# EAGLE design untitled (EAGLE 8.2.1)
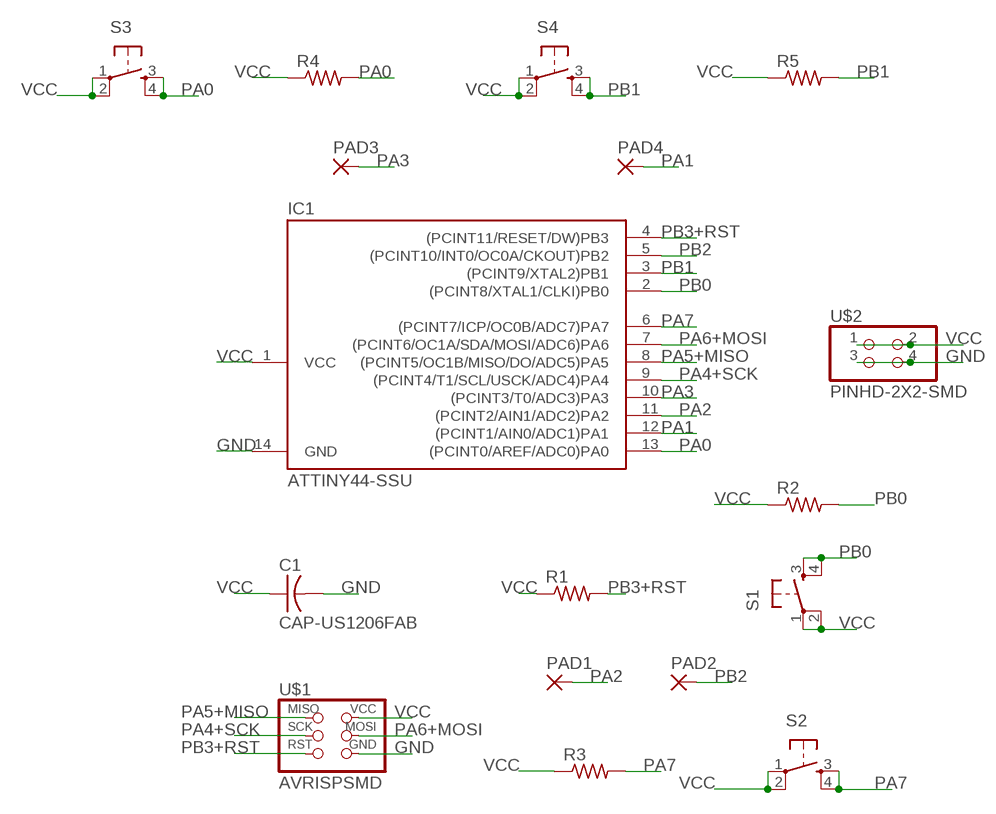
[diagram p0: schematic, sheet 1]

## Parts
C1  CAP-US1206FAB  [C1206FAB]
IC1  ATTINY44-SSU  [SOIC14]
PAD1  SMD2  [SMD1,27-2,54]
PAD2  SMD2  [SMD1,27-2,54]
PAD3  SMD2  [SMD1,27-2,54]
PAD4  SMD2  [SMD1,27-2,54]
R1  RES-US1206FAB  [R1206FAB]
R2  RES-US1206FAB  [R1206FAB]
R3  RES-US1206FAB  [R1206FAB]
R4  RES-US1206FAB  [R1206FAB]
R5  RES-US1206FAB  [R1206FAB]
S1  6MM_SWITCH6MM_SWITCH  [6MM_SWITCH]
S2  6MM_SWITCH6MM_SWITCH  [6MM_SWITCH]
S3  6MM_SWITCH6MM_SWITCH  [6MM_SWITCH]
S4  6MM_SWITCH6MM_SWITCH  [6MM_SWITCH]
U$1  AVRISPSMD  [2X03SMD]
U$2  PINHD-2X2-SMD  [2X02SMD]

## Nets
GND: C1.2 IC1.14(GND) U$1.6(GND) U$2.3 U$2.4
PA0: IC1.13((PCINT0/AREF/ADC0)PA0) R4.2 S3.3(S) S3.4(S1)
PA1: IC1.12((PCINT1/AIN0/ADC1)PA1) PAD4.1(P)
PA2: IC1.11((PCINT2/AIN1/ADC2)PA2) PAD1.1(P)
PA3: IC1.10((PCINT3/T0/ADC3)PA3) PAD3.1(P)
PA4+SCK: IC1.9((PCINT4/T1/SCL/USCK/ADC4)PA4) U$1.3(SCK)
PA5+MISO: IC1.8((PCINT5/OC1B/MISO/DO/ADC5)PA5) U$1.1(MISO)
PA6+MOSI: IC1.7((PCINT6/OC1A/SDA/MOSI/ADC6)PA6) U$1.4(MOSI)
PA7: IC1.6((PCINT7/ICP/OC0B/ADC7)PA7) R3.2 S2.3(S) S2.4(S1)
PB0: IC1.2((PCINT8/XTAL1/CLKI)PB0) R2.2 S1.3(S) S1.4(S1)
PB1: IC1.3((PCINT9/XTAL2)PB1) R5.2 S4.3(S) S4.4(S1)
PB2: IC1.5((PCINT10/INT0/OC0A/CKOUT)PB2) PAD2.1(P)
PB3+RST: IC1.4((PCINT11/RESET/DW)PB3) R1.2 U$1.5(RST)
VCC: C1.1 IC1.1(VCC) R1.1 R2.1 R3.1 R4.1 R5.1 S1.1(P) S1.2(P1) S2.1(P) S2.2(P1) S3.1(P) S3.2(P1) S4.1(P) S4.2(P1) U$1.2(VCC) U$2.1 U$2.2

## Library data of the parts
C1 = fab:CAP-US
IC1 = fab:ATTINY44
PAD1-PAD4 = wirepad:SMD2: SMD PAD
R1-R5 = fab:RES-US: Resistor (US Symbol)
S1-S4 = fab:6MM_SWITCH: OMRON SWITCH
U$1 = fab:AVRISP
U$2 = fab:PINHD-2X2-SMD

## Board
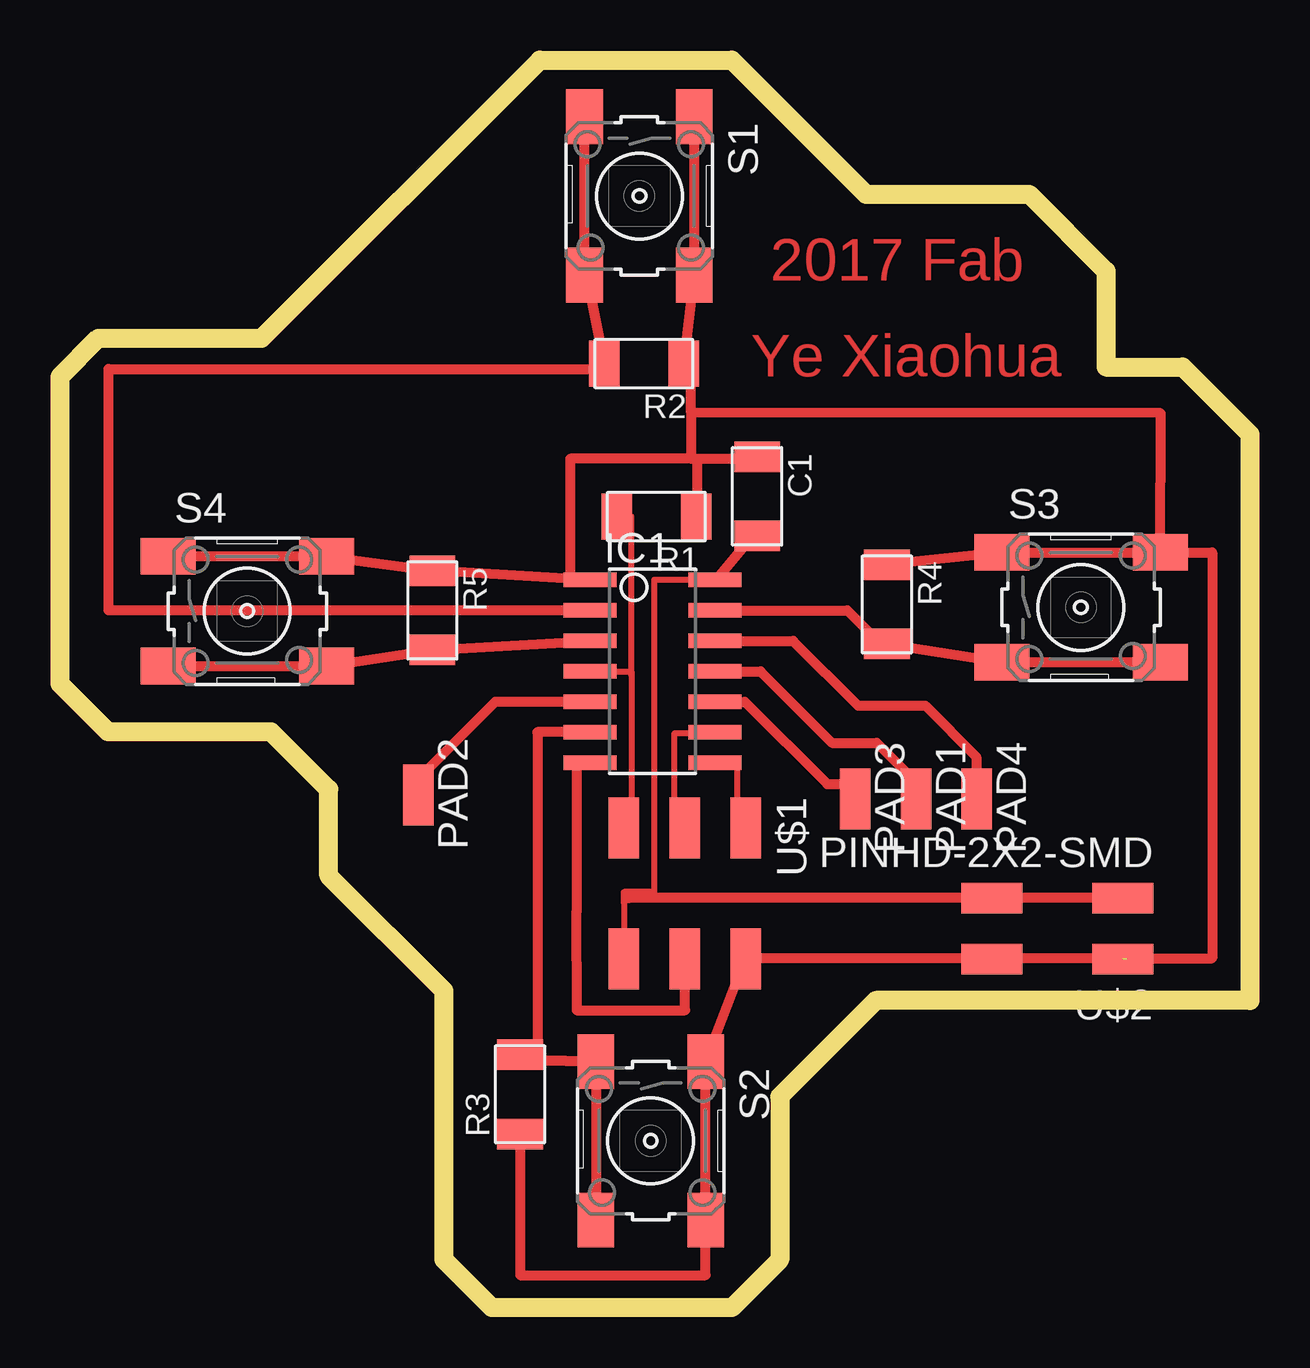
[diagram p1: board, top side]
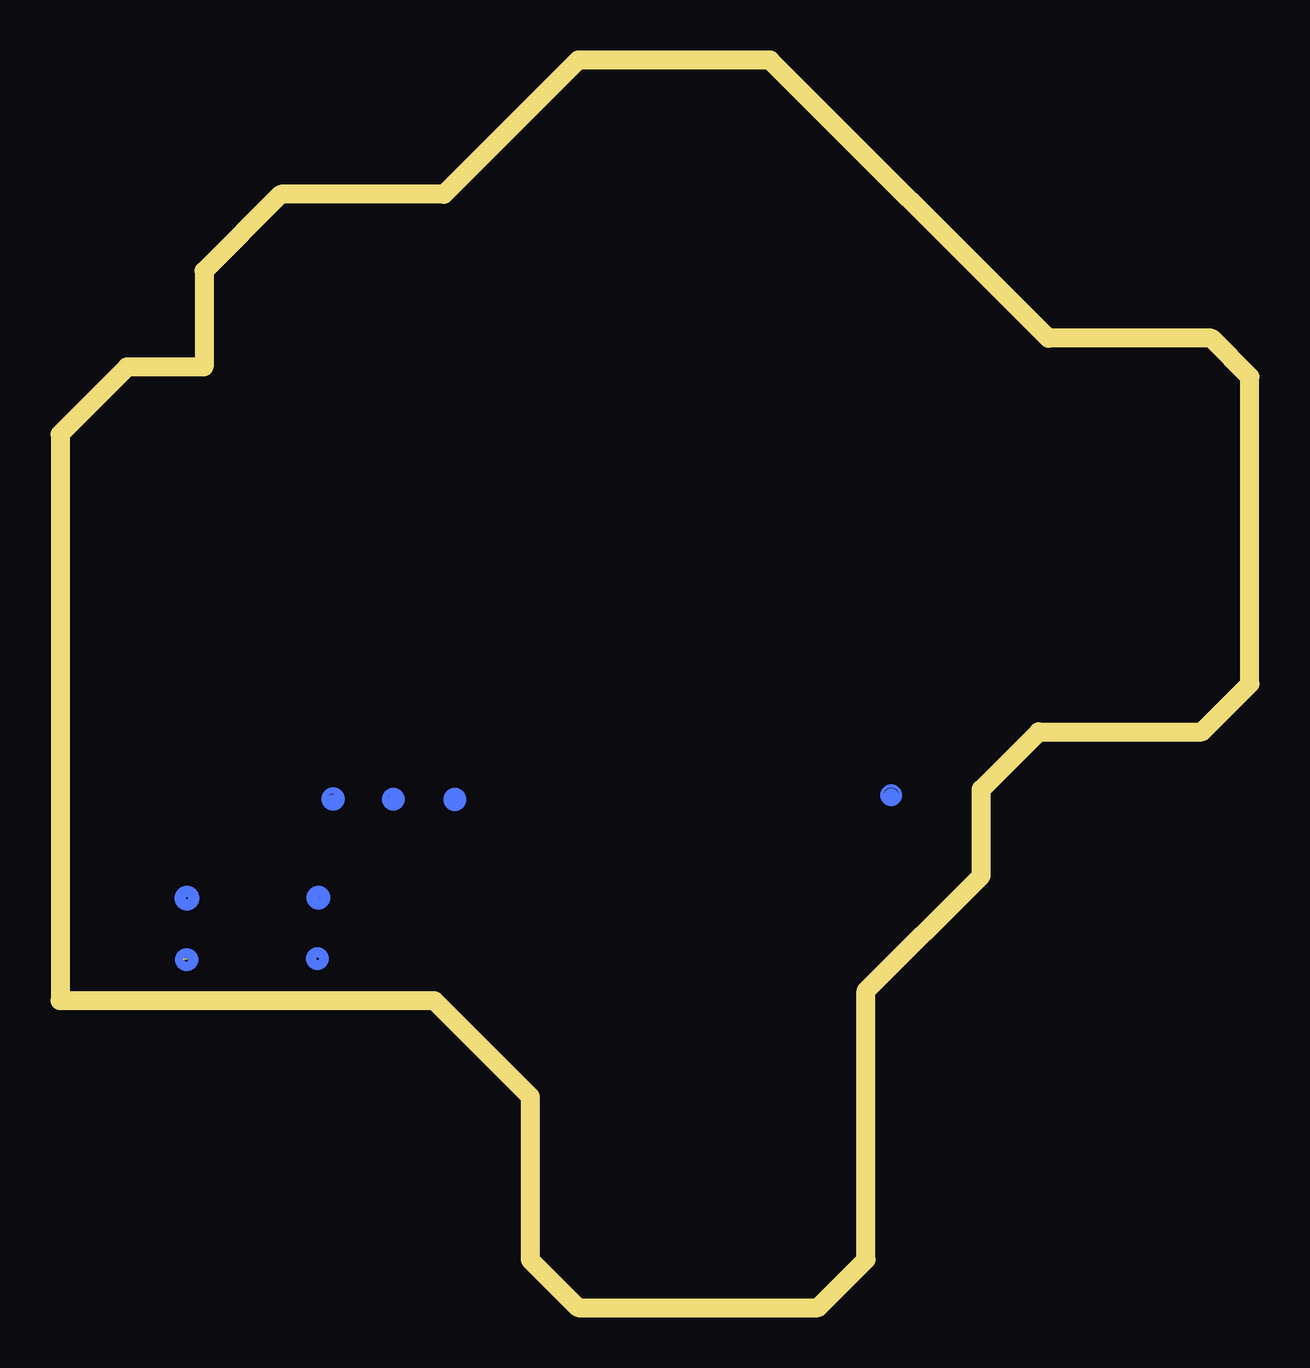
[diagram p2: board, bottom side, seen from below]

Size 49.6 x 52 mm. Coordinates in mm from the lower left corner, seen from the top.
Outline: 1.6,40.4 8.4,40.4 20,52 28,52 33.6,46.4 40.4,46.4 43.6,43.2 43.6,39.2 46.8,39.2 49.6,36.4 49.6,12.8 34,12.8 30,8.8 30,2 28,0 18,0 16,2 16,13.2 11.2,18 11.2,21.6 8.8,24 2,24 0,26 0,38.8 1.6,40.4
Copper layers (1*16): Top 0.035mm / dielectric 1.5mm / Bottom 0.035mm
Design rules "default": minimum track width 10mil, minimum drill 24mil, track to track 8mil, track to pad 8mil, pad to pad 8mil, via to via 8mil, smd to smd 8mil, copper to edge 40mil, drill to drill 8mil, minimum pad ring 10mil, minimum via ring 8mil, stop-mask expansion 4mil, vias tented up to drill 0mil, thermal gap 10mil

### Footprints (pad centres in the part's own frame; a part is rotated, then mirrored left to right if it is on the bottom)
C1206FAB = smd 1.27 x 1.905: 1 -1.651,0; 2 1.651,0
SOIC14 = smd 0.61 x 2.21: 1 -3.81,-2.603; 2 -2.54,-2.603; 3 -1.27,-2.603; 4 0,-2.603; 5 1.27,-2.603; 6 2.54,-2.603; 7 3.81,-2.603; 8 3.81,2.603; 9 2.54,2.603; 10 1.27,2.603; 11 0,2.603; 12 -1.27,2.603; 13 -2.54,2.603; 14 -3.81,2.603
SMD1,27-2,54 = smd 1.27 x 2.54: 1 0,0
R1206FAB = smd 1.27 x 1.905: 1 -1.651,0; 2 1.651,0
6MM_SWITCH = smd 2.286 x 1.524: 1 -3.302,2.286; 2 3.302,2.286; 3 -3.302,-2.286; 4 3.302,-2.286
2X03SMD = smd 2.54 x 1.27: 1 -2.54,2.54; 2 2.92,2.54; 3 -2.54,0; 4 2.92,0; 5 -2.54,-2.54; 6 2.92,-2.54
2X02SMD = smd 2.54 x 1.27: 1 -2.54,1.27; 2 2.92,1.27; 3 -2.54,-1.27; 4 2.92,-1.27

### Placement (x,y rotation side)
C1  29.06,33.81 270 top
IC1  24.7,26.52 270 top
PAD1  35.69,21.19 180 top
PAD2  14.94,21.36 180 top
PAD3  33.14,21.2 180 top
PAD4  38.21,21.19 180 top
R1  24.86,32.97 180 top
R2  24.34,39.35 180 top
R3  19.18,8.89 90 top
R4  34.47,29.31 270 top
R5  15.52,29.06 270 top
S1  24.15,46.33 270 top
S2  24.62,6.95 270 top
S3  42.56,29.19 0 top
S4  7.81,29.03 0 top
U$1  26.05,17.46 270 top
U$2  41.76,15.8 180 top

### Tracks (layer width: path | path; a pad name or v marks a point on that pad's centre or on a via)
GND
  Top 0.254: C1.2 28.84,32.13 | 27.39,30.38 27.3,30.49 IC1.14 24.76,30.33 24.76,17.32 23.51,17.32 23.51,16.87 | 23.51,16.87 U$1.6 | 23.71,17.07 23.51,16.87
  Top 0.406: 28.84,32.13 27.39,30.38 | U$2.3 U$2.4 23.71,17.07
PA0
  Top 0.254: 33.97,27.91 34.22,27.91 R4.2
  Top 0.406: S3.4 S3.3 R4.2 | IC1.13 32.82,29.06 33.97,27.91
PA1
  Top 0.254: 38.2,21.21 PAD4.1
  Top 0.406: IC1.12 30.56,27.79 33.26,25.08 36.06,25.08 38.2,22.95 38.2,21.21
PA2
  Top 0.254: 35.33,22.26 35.33,21.55 PAD1.1
  Top 0.406: IC1.11 29.2,26.52 32.18,23.54 34.05,23.54 35.33,22.26
PA3
  Top 0.254: 33.2,21.81 33.22,21.79 33.22,21.27 PAD3.1
  Top 0.406: IC1.10 28.55,25.25 31.98,21.81 33.2,21.81
PA4+SCK
  Top 0.254: U$1.3 25.62,20 25.62,23.95 27.3,23.95 IC1.9
PA5+MISO
  Top 0.254: IC1.8 28.22,22.71 28.22,20.41 28.59,20.41 U$1.1
PA6+MOSI
  Top 0.254: IC1.7 21.52,22.71 | 21.53,16.48 21.52,16.48
  Top 0.406: 21.52,22.71 21.53,16.48 | 21.52,16.48 21.53,12.39 26.06,12.39 U$1.4
PA7
  Top 0.254: 19.9,10.29 21.06,10.29 | 22.34,10.29 S2.3 | 19.18,10.29 R3.2
  Top 0.406: S2.3 S2.4 | IC1.6 19.9,23.98 19.9,10.29 | 22.34,10.29 21.06,10.29 19.18,10.29
PB0
  Top 0.254: 21.87,43.55 S1.4 | 22.69,39.12 R2.2
  Top 0.406: S1.3 21.87,43.55 R2.2 | IC1.2 2.02,29.06 2.02,39.12 22.69,39.12
PB1
  Top 0.406: S4.3 S4.4 R5.2 IC1.3
PB2
  Top 0.254: 15.37,22.47 15.37,21.78 PAD2.1
  Top 0.406: IC1.5 18.14,25.25 15.37,22.47
PB3+RST
  Top 0.254: R1.2 23.82,32.97 23.82,26.36 | 23.82,26.36 23.82,20.76 23.51,20.76 U$1.5 | IC1.4 23.82,26.52 23.82,26.36
VCC  (1 unrouted)
  Top 0.254: 28.54,14.54 U$1.2 28.59,14.55 | 26.51,32.92 R1.1 26.57,32.97 | 29.08,35.39 C1.1 | 26.31,35.39 26.57,35.39 | 21.28,30.34 IC1.1 | R2.1 26.31,39.35 | R3.1 | U$2.2 44.47,14.53 44.49,14.55
  Top 0.406: 26.57,32.97 26.57,35.39 29.08,35.39 | 21.28,30.34 21.28,35.39 26.31,35.39 26.31,37.31 | R4.1 S3.1 S3.2 | S1.1 S1.2 R2.1 | IC1.1 R5.1 S4.2 S4.1 | 26.31,37.31 26.31,39.35 | S3.2 45.89,37.28 26.31,37.31 | 28.54,14.54 S2.1 S2.2 26.91,1.35 19.18,1.35 R3.1 | S3.2 48.03,31.47 48.03,14.55 44.49,14.55 28.59,14.55
(copper drawn outside any net)
  shapes: Bottom circle x29

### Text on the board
Top: 2017 Fab | Ye Xiaohua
